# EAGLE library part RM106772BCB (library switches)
Rotary Switch 6 Position SP6T 500mA (DC) 24VDC Through Hole
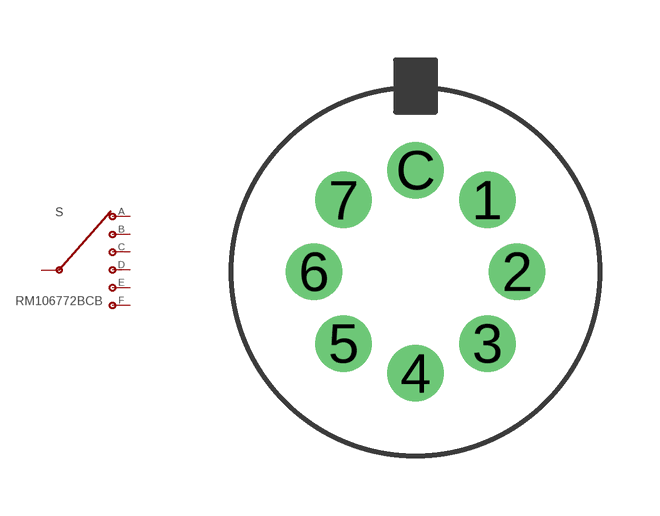
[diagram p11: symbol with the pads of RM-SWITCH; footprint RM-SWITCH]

Designator prefix S

## RM106772BCB (DIGIKEY: CKN10703-ND)  [RM-SWITCH]
1  A
2  B
3  C
4  D
5  E
6  F
C  INPUT

## Footprint RM-SWITCH (pad centres in mm)
drill 0.9: 1 1.796,1.796; 2 2.54,0; 3 1.796,-1.796; 4 0,-2.54; 5 -1.796,-1.796; 6 -2.54,0; 7 -1.796,1.796; C 0,2.54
